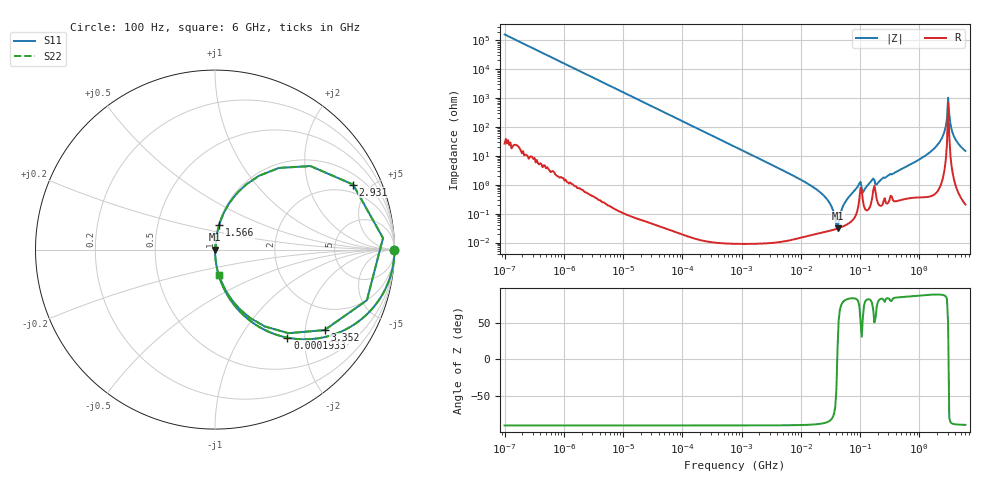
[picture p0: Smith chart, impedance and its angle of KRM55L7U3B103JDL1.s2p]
!Murata Part Number: KRM55L7U3B103JDL1
!These Parameters are Measured in Series Mode Connection
!Data Generated on Jan 08, 2026
!  o--ll--o
!Port1  Port2
!  o------o
!Operation Temp=25[degC], DC Bias Voltage=0[V]
!Freq. Start=100[Hz] Stop=6[GHz] 401[Steps]
# Hz S RI R 50
!Freq.(Hz) S11(Real) S11(Imag) S21(Real) S21(Imag) S12(Real) S12(Imag) S22(Real) S22(Imag)
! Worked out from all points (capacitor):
!   401 points, 100 Hz to 6 GHz, reference 50 ohm
!   read as one part in series: C = 10 nF near 109 Hz
!   lowest |Z| = 31.5 mohm at 41.66 MHz (marker M1)
!   series resonance near 41.25 MHz, so ESL is about 1.5 nH
!   S11 on the Smith chart (normalised r, x): 100 Hz: open; 193.3 kHz: 1.00, -1.65; 1.566 GHz: 1.01, +0.28; 2.931 GHz: 1.50, +3.93; 3.352 GHz: 1.21, -2.54; 6 GHz: 1.00, -0.30
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100  1 -0.000629  5e-07 0.000629  5e-07 0.000629  1 -0.000629
2008  0.9998 -0.0126  0.00016 0.0126  0.00016 0.0126  0.9998 -0.0126
40335  0.9396 -0.2382  0.0604 0.2382  0.0604 0.2382  0.9396 -0.2382
193316  0.4038 -0.4906  0.5962 0.4906  0.5962 0.4906  0.4038 -0.4906
774597  0.0405 -0.197  0.9595 0.197  0.9595 0.197  0.0405 -0.197
1.555665e7  0.00026 -0.00873  0.9997 0.00873  0.9997 0.00873  0.00026 -0.00873
2.784235e7  0.000252 -0.0031  0.9997 0.0031  0.9997 0.0031  0.000252 -0.0031
4.165952e7  0.000305 7.81e-05  0.9997 -7.81e-05  0.9997 -7.81e-05  0.000305 7.81e-05
5.699437e7  0.000405 0.00261  0.9996 -0.00261  0.9996 -0.00261  0.000405 0.00261
9.326766e7  0.00183 0.00911  0.9982 -0.00911  0.9982 -0.00911  0.00183 0.00911
1.166697e8  0.00182 0.00609  0.9982 -0.00609  0.9982 -0.00609  0.00182 0.00609
1.596157e8  0.00351 0.0141  0.9965 -0.0141  0.9965 -0.0141  0.00351 0.0141
1.996653e8  0.00247 0.0113  0.9975 -0.0113  0.9975 -0.0113  0.00247 0.0113
3.124326e8  0.00333 0.0221  0.9967 -0.0221  0.9967 -0.0221  0.00333 0.0221
1.565993e9  0.0234 0.1375  0.9766 -0.1375  0.9766 -0.1375  0.0234 0.1375
2.34314e9  0.1289 0.3209  0.8711 -0.3209  0.8711 -0.3209  0.1289 0.3209
2.679998e9  0.356 0.455  0.644 -0.455  0.644 -0.455  0.356 0.455
2.931063e9  0.7693 0.3624  0.2307 -0.3624  0.2307 -0.3624  0.7693 0.3624
3.352442e9  0.6102 -0.4485  0.3898 0.4485  0.3898 0.4485  0.6102 -0.4485
3.666503e9  0.2783 -0.4285  0.7217 0.4285  0.7217 0.4285  0.2783 -0.4285
4.009986e9  0.1435 -0.337  0.8565 0.337  0.8565 0.337  0.1435 -0.337
6e9  0.0233 -0.144  0.9767 0.144  0.9767 0.144  0.0233 -0.144
